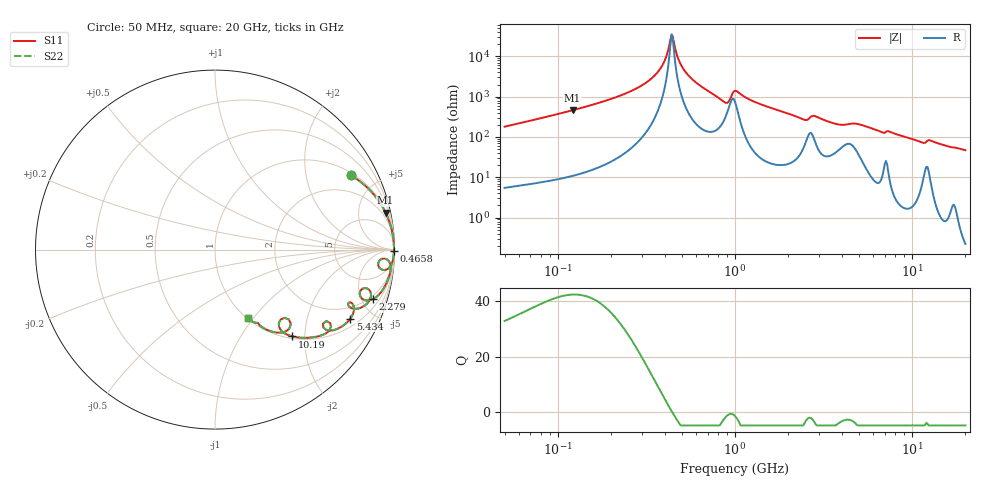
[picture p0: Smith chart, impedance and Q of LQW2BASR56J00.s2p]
!Murata Part Number: LQW2BASR56J00
!These Parameters are Measured in Series Mode Connection
!  o--[Z]--o
!Port1  Port2
!  o-------o
!Freq. Start=50[MHz] Stop=20[GHz], 401[Steps]
# Hz S RI R 50
!Freq.(Hz) S11(Real) S11(Imag) S21(Real) S21(Imag) S12(Real) S12(Imag) S22(Real) S22(Imag)
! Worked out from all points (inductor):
!   401 points, 50 MHz to 20 GHz, reference 50 ohm
!   read as one part in series: L = 563 nH near 51.52 MHz
!   highest Q = 42.4 at 121 MHz (marker M1), where L = 605 nH
!   self-resonance near 438.7 MHz
!   S11 on the Smith chart (normalised r, x): 50 MHz: 1.11, +3.60; 465.8 MHz: open; 2.279 GHz: 1.64, -6.10; 5.434 GHz: 1.36, -3.69; 10.19 GHz: 1.04, -1.74; 20 GHz: 1.00, -0.94
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5e7  0.7575 0.4137  0.2425 -0.4137  0.2425 -0.4137  0.7575 0.4137
1.209968e8  0.9505 0.2055  0.0495 -0.2055  0.0495 -0.2055  0.9505 0.2055
1.364002e8  0.9616 0.1807  0.0384 -0.1807  0.0384 -0.1807  0.9616 0.1807
2.636584e8  0.9924 0.0692  0.00756 -0.0692  0.00756 -0.0692  0.9924 0.0692
3.251725e8  0.9958 0.0401  0.00425 -0.0401  0.00425 -0.0401  0.9958 0.0401
3.721004e8  0.9968 0.0222  0.00315 -0.0222  0.00315 -0.0222  0.9968 0.0222
4.010383e8  0.9971 0.0123  0.00286 -0.0123  0.00286 -0.0123  0.9971 0.0123
4.387496e8  0.9972 0.000459  0.00283 -0.000459  0.00283 -0.000459  0.9972 0.000459
4.520922e8  0.9971 -0.00353  0.00289 0.00353  0.00289 0.00353  0.9971 -0.00353
4.658406e8  0.997 -0.00754  0.003 0.00754  0.003 0.00754  0.997 -0.00754
5.251442e8  0.9961 -0.0239  0.00389 0.0239  0.00389 0.0239  0.9961 -0.0239
6.673612e8  0.9907 -0.0607  0.00932 0.0607  0.00932 0.0607  0.9907 -0.0607
8.870719e8  0.9255 -0.1094  0.0745 0.1094  0.0745 0.1094  0.9255 -0.1094
1e9  0.9597 -0.0559  0.0403 0.0559  0.0403 0.0559  0.9597 -0.0559
1.329223e9  0.9734 -0.1373  0.0266 0.1373  0.0266 0.1373  0.9734 -0.1373
2.279204e9  0.8805 -0.276  0.1195 0.276  0.1195 0.276  0.8805 -0.276
2.728004e9  0.8494 -0.2173  0.1506 0.2173  0.1506 0.2173  0.8494 -0.2173
3.626126e9  0.7857 -0.3299  0.2143 0.3299  0.2143 0.3299  0.7857 -0.3299
5.433528e9  0.754 -0.3846  0.246 0.3846  0.246 0.3846  0.754 -0.3846
7.442007e9  0.6391 -0.4469  0.3609 0.4469  0.3609 0.4469  0.6391 -0.4469
1.019291e10  0.4315 -0.4839  0.5685 0.4839  0.5685 0.4839  0.4315 -0.4839
2e10  0.1823 -0.3837  0.8177 0.3837  0.8177 0.3837  0.1823 -0.3837
